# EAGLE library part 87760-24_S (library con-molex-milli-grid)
HEADER
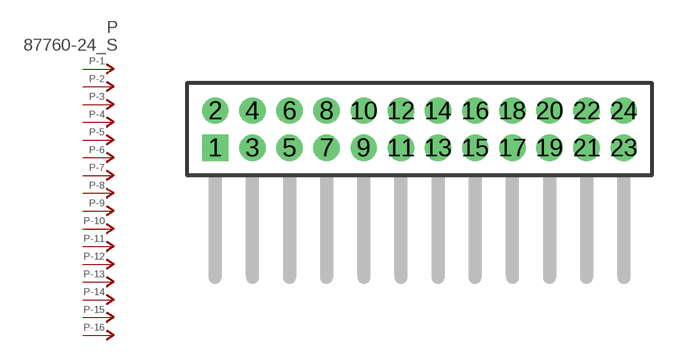
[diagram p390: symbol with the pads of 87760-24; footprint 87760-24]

Designator prefix P; gates -1=P-NV -2=P-N -3=P-N -4=P-N -5=P-N -6=P-N -7=P-N -8=P-N -9=P-N -10=P-N -11=P-N -12=P-N -13=P-N -14=P-N -15=P-N -16=P-N -17=P-N -18=P-N -19=P-N -20=P-N -21=P-N -22=P-N -23=P-N -24=P-N

## 87760-24_S  [87760-24]
1  -1:P  pas
2  -2:P  pas
3  -3:P  pas
4  -4:P  pas
5  -5:P  pas
6  -6:P  pas
7  -7:P  pas
8  -8:P  pas
9  -9:P  pas
10  -10:P  pas
11  -11:P  pas
12  -12:P  pas
13  -13:P  pas
14  -14:P  pas
15  -15:P  pas
16  -16:P  pas
17  -17:P  pas
18  -18:P  pas
19  -19:P  pas
20  -20:P  pas
21  -21:P  pas
22  -22:P  pas
23  -23:P  pas
24  -24:P  pas

## Footprint 87760-24 (pad centres in mm)
HEADER Dual Row, Right Angle
drill 0.914 square: 1 -11,-1
drill 0.914: 2 -11,1; 3 -9,-1; 4 -9,1; 5 -7,-1; 6 -7,1; 7 -5,-1; 8 -5,1; 9 -3,-1; 10 -3,1; 11 -1,-1; 12 -1,1; 13 1,-1; 14 1,1; 15 3,-1; 16 3,1; 17 5,-1; 18 5,1; 19 7,-1; 20 7,1; 21 9,-1; 22 9,1; 23 11,-1; 24 11,1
